(* Logix 5000 AddOnInstructionDefinition export RTA_SCNDR_Heartbeat_AOI; software revision 32.00 *)

ADD_ON_INSTRUCTION RTA_SCNDR_Heartbeat_AOI   (* revision 1.0, vendor Real Time Automation, Inc. *)
// RTA's 435NBX heartbeat handshaking
VAR_IN_OUT
   DataIn : INT; {required}
   DataOut : BOOL; {required}
END_VAR
VAR
   Previous_Value : INT; {access None}
   Number_of_Times_Inactive : INT; {access None}
END_VAR

ROUTINE Logic   (* ladder *)
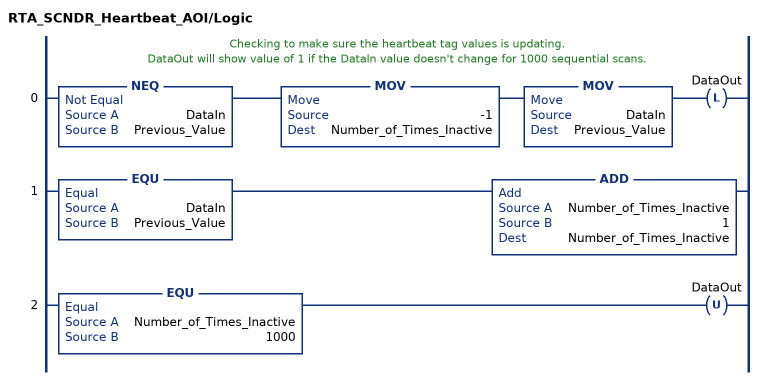
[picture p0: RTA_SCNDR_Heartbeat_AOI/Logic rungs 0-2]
   // Checking to make sure the heartbeat tag values is updating.
   // DataOut will show value of 1 if the DataIn value doesn't change for 1000 sequential scans.
   0: NEQ(DataIn,Previous_Value)MOV(-1,Number_of_Times_Inactive)MOV(DataIn,Previous_Value)OTL(DataOut);
   1: EQU(DataIn,Previous_Value)ADD(Number_of_Times_Inactive,1,Number_of_Times_Inactive);
   2: EQU(Number_of_Times_Inactive,1000)OTU(DataOut);
END_ROUTINE
END_ADD_ON_INSTRUCTION
